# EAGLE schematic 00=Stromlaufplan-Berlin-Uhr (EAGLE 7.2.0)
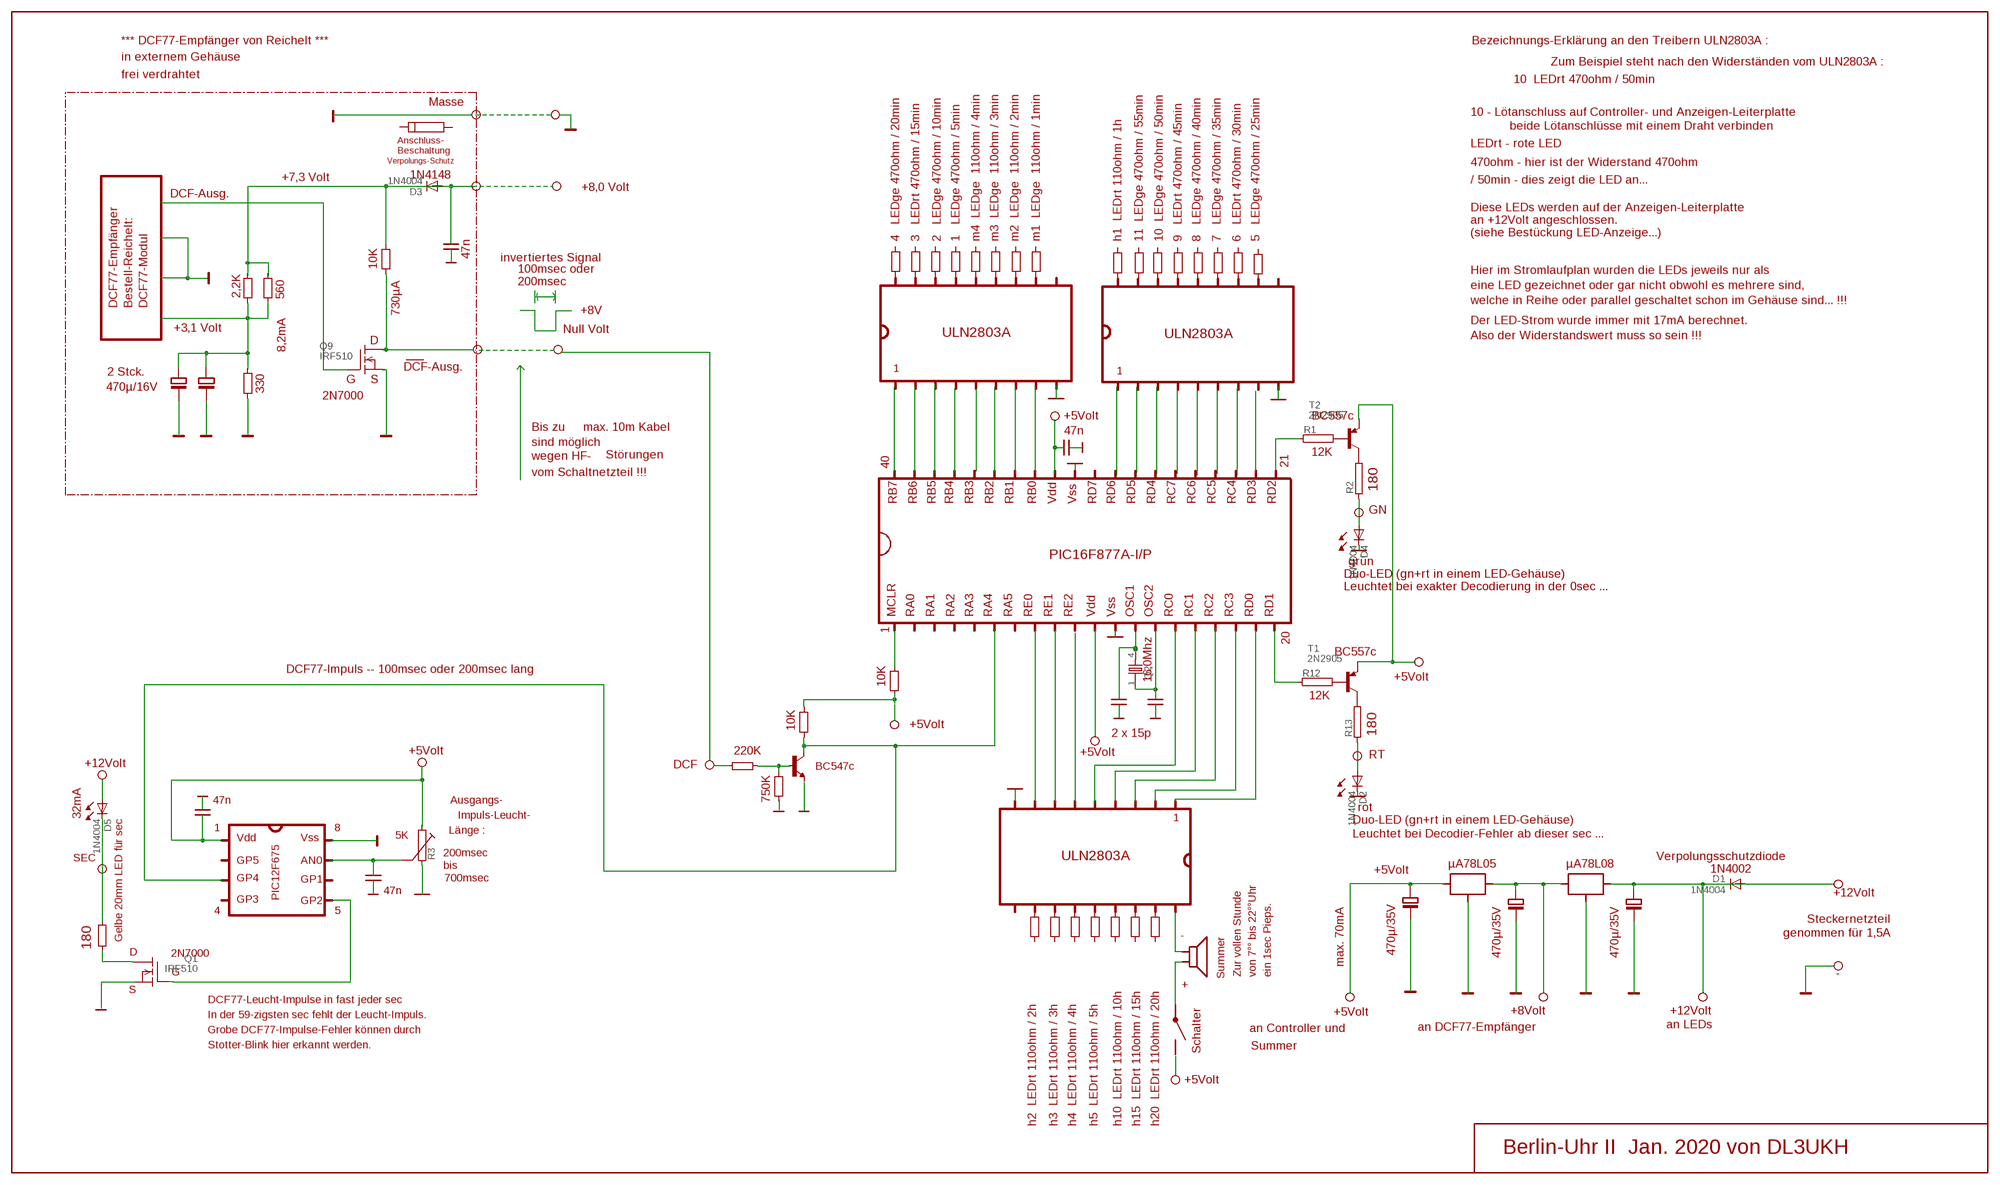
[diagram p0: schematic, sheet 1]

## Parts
D1  1N4004  [DO41-10]
D2  1N4004  [DO41-10]
D3  1N4004  [DO41-10]
D4  1N4004  [DO41-10]
D5  1N4004  [DO41-10]
Q1  IRF510  [TO220]
Q2  86SMX  [86SMX]
Q9  IRF510  [TO220]
R1  RHS10  [HS10]
R2  RHS10  [HS10]
R3  RHS10  [HS10]
R12  RHS10  [HS10]
R13  RHS10  [HS10]
T1  2N2905  [TO5]
T2  2N2905  [TO5]

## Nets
N$9: R12.2 T1.2(B)
N$14: Q2.4
N$15: Q2.1
N$22: D2.C
N$23: Q9.2(D)
N$48: D1.A D1.C
N$68: Q9.3(S)
N$70: Q9.1(G)
N$77: D3.A D3.C
N$78: R13.2 T1.3(C)
N$80: D2.A R13.1
N$81: R1.2 T2.2(B)
N$82: D4.C
N$83: R2.2 T2.3(C)
N$84: D4.A R2.1
N$87: T1.1(E)
N$92: R3.2
N$97: Q1.1(G)
N$98: Q1.3(S)
N$100: R3.1
N$103: D5.A
N$104: Q1.2(D)
N$108: D5.C
Unconnected: R1.1 R12.1 T2.1(E)

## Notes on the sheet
- *** DCF77-Empfänger von Reichelt *** | Bezeichnungs-Erklärung an den Treibern ULN2803A :
- Zum Beispiel steht nach den Widerständen vom ULN2803A :
- in externem Gehäuse
- 10  LEDrt 470ohm / 50min
- frei verdrahtet
- Masse
- 10 - Lötanschluss auf Controller- und Anzeigen-Leiterplatte
- beide Lötanschlüsse mit einem Draht verbinden
- Anschluss-
- LEDrt - rote LED
- Beschaltung
- Verpolungs-Schutz
- 470ohm - hier ist der Widerstand 470ohm
- +7,3 Volt | 1N4148
- +8,0 Volt | / 50min - dies zeigt die LED an...
- DCF-Ausg.
- Diese LEDs werden auf der Anzeigen-Leiterplatte
- an +12Volt angeschlossen.
- 47n | (siehe Bestückung LED-Anzeige...)
- 4   LEDge 470ohm / 20min | 3   LEDrt 470ohm / 15min | 2   LEDge 470ohm / 10min | 1   LEDge 470ohm / 5min | m4  LEDge  110ohm / 4min | m3  LEDge  110ohm / 3min | m2  LEDge  110ohm / 2min | m1  LEDge  110ohm / 1min | h1  LEDrt 110ohm / 1h | 11  LEDge 470ohm / 55min | 10  LEDge 470ohm / 50min | 9   LEDrt 470ohm / 45min | 8   LEDge 470ohm / 40min | 7   LEDge 470ohm / 35min | 6   LEDrt 470ohm / 30min | 5   LEDge 470ohm / 25min
- invertiertes Signal
- 10K
- 100msec oder | Hier im Stromlaufplan wurden die LEDs jeweils nur als
- 200msec
- eine LED gezeichnet oder gar nicht obwohl es mehrere sind,
- 2,2K | 560
- welche in Reihe oder parallel geschaltet schon im Gehäuse sind... !!!
- DCF77-Empfänger | Bestell-Reichelt: | DCF77-Modul
- 730µA | +8V
- Der LED-Strom wurde immer mit 17mA berechnet.
- +3,1 Volt | Null Volt
- ULN2803A | ULN2803A | Also der Widerstandswert muss so sein !!!
- D
- 8,2mA
- DCF-Ausg. | 1
- 2 Stck. | 1
- G | S
- 470µ/16V | 330
- 2N7000
- +5Volt | BC557c
- 47n
- Bis zu | max. 10m Kabel
- sind möglich | 12K
- wegen HF- | Störungen
- 40 | 21
- vom Schaltnetzteil !!!
- 180
- RB7 | RB6 | RB5 | RB4 | RB3 | RB2 | RB1 | RB0 | Vdd | Vss | RD7 | RD6 | RD5 | RD4 | RC7 | RC6 | RC5 | RC4 | RD3 | RD2
- GN
- PIC16F877A-I/P
- grün
- Duo-LED (gn+rt in einem LED-Gehäuse)
- Leuchtet bei exakter Decodierung in der 0sec ...
- MCLR | RA0 | RA1 | RA2 | RA3 | RA4 | RA5 | RE0 | RE1 | RE2 | Vdd | Vss | OSC1 | OSC2 | RC0 | RC1 | RC2 | RC3 | RD0 | RD1
- 1
- 16,0Mhz
- 20
- BC557c
- DCF77-Impuls -- 100msec oder 200msec lang | 10K
- +5Volt
- 12K
- 10K
- +5Volt
- 2 x 15p
- 180
- +5Volt | 220K
- +12Volt | +5Volt | RT
- DCF
- BC547c
- 47n | Ausgangs- | 750K
- rot
- 32mA | Impuls-Leucht- | 1
- Duo-LED (gn+rt in einem LED-Gehäuse)
- 1 | 8 | Länge :
- 5K | Leuchtet bei Decodier-Fehler ab dieser sec ...
- Vdd | Vss
- 200msec
- SEC | ULN2803A | Verpolungsschutzdiode
- GP5 | AN0 | +5Volt
- bis | µA78L05 | µA78L08
- 1N4002
- GP4 | GP1 | 700msec
- 47n
- +12Volt
- GP3 | PIC12F675
- GP2
- 4 | 5
- Steckernetzteil
- -
- Summer | genommen für 1,5A
- Gelbe 20mm LED für sec
- 180
- D | 2N7000 | 470µ/35V | 470µ/35V | 470µ/35V
- max. 70mA
- G | Zur vollen Stunde | von 7°° bis 22°°Uhr | ein 1sec Pieps. | -
- +
- S
- DCF77-Leucht-Impulse in fast jeder sec
- +5Volt | +8Volt | +12Volt
- In der 59-zigsten sec fehlt der Leucht-Impuls.
- an DCF77-Empfänger | an LEDs
- Grobe DCF77-Impulse-Fehler können durch | an Controller und
- Stotter-Blink hier erkannt werden. | Summer
- Schalter
- +5Volt
- h2  LEDrt 110ohm / 2h | h3  LEDrt 110ohm / 3h | h4  LEDrt 110ohm / 4h | h5  LEDrt 110ohm / 5h | h10  LEDrt 110ohm / 10h | h15  LEDrt 110ohm / 15h | h20  LEDrt 110ohm / 20h
- Berlin-Uhr II  Jan. 2020 von DL3UKH

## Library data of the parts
D1-D5 = diode:1N4004: DIODE
Q1 Q9 = transistor-fet:IRF510: N-Channel Enhancement MOSFET (HEXFET); 100V; 5,6A; 0,54Ohm
Q2 = crystal:86SMX: CRYSTAL
R1-R3 R12 R13 = resistor-power:R: Power Resitor
T1 T2 = transistor-pnp:2N2905: PNP Transistor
